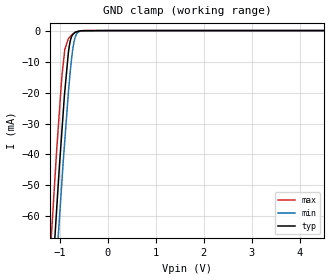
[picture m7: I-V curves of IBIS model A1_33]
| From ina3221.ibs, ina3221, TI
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|   A1 input model
[Model]   A1_33
Model_type   Input
Vinl = 0.99   |min, GND -0.5 V
Vinh = 2.31   |max. V+ 6 V
|   typ   min   max
|   (nom PVT)   (Fast PVT)   (slow PVT)
C_comp   5.836E-13   5.547E-13   6.340E-13
| Where   nom PVT is  Nominal Process, 3.3V, 25C
|   Fast PVT is Strong Process, 3.6V, -40C
|   Slow PVT is Weak Process, 3.0V, 85C
|C_comp - from L-C Tank method, L = 1nH, peak frequency
[Model Spec]
| variable   typ   min   max
Vinl   0.99   0.9   1.08
Vinh   2.31   2.1   2.52
|Vinl = 0.3 x V+, Vinh = 0.7 x V+
[Voltage Range]   3.3   3   3.6
|Ambient Temperature Range   27   85   -40
[Temperature Range]   30   88   -40
[Power Clamp Reference]   3.3   3   3.6
[GND Clamp Reference]   0   0   0
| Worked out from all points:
|   GND clamp passes 1 mA (typ) near -0.71 V on its own axis
[GND Clamp]
|   Voltage   I(typ)   I(min)   I(max)
-3.3V     -649.7mA   -656.5mA   -642.6mA
-1.178V   -84.67mA   -101.3mA   -66.35mA
-1.073V   -59.17mA   -75.54mA   -40.21mA
-1.064V   -56.98mA   -73.4mA    -37.96mA
-1.016V   -45.31mA   -62.27mA   -27.45mA
-958.6mV  -32.61mA   -48.9mA    -14.93mA
-897.4mV  -19.64mA   -35.5mA    -6.08mA
-803.9mV  -5.045mA   -16.68mA   -2.273mA
-735.4mV  -1.334mA   -6.489mA   -1.2mA
-683.6mV  -535.5uA   -2.3mA     -623.7uA
-573.6mV  -64.07uA   -170.3uA   -127.6uA
6.59V     0A         0A         0A
[POWER Clamp]
|   SCR cell for ESD function. Effects occurr above VDD x 2
|   Voltage   I(typ)   I(min)   I(max)
-3.3V     0A         0A         0A
0V        0A         0A         0A
6.6V      0A         0A         0A
